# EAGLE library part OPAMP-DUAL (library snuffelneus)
Operational Amplifier
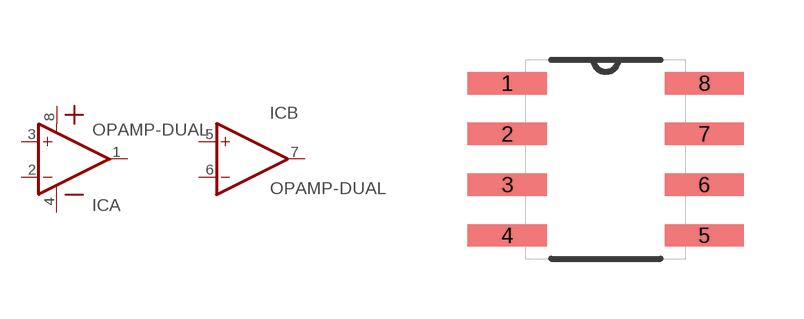
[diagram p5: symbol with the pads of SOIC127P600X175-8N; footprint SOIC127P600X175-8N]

Designator prefix IC; gates B=OP-AMP A=OP-AMP+-

## OPAMP-DUAL  [SOIC127P600X175-8N]
1  A:OUT  out
2  A:-IN  in
3  A:+IN  in
4  A:GND  pwr
5  B:+IN  in
6  B:-IN  in
7  B:OUT  out
8  A:VDD  pwr

## Footprint SOIC127P600X175-8N (pad centres in mm)
smd 1.981 x 0.559: 1 -2.464,1.905; 2 -2.464,0.635; 3 -2.464,-0.635; 4 -2.464,-1.905; 5 2.464,-1.905; 6 2.464,-0.635; 7 2.464,0.635; 8 2.464,1.905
